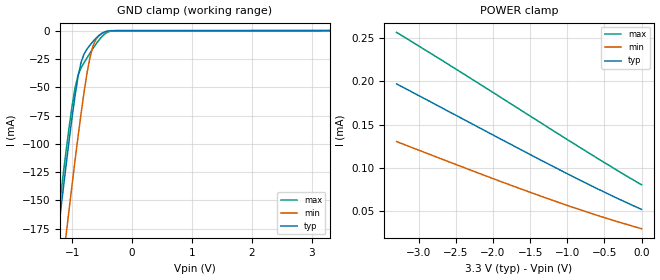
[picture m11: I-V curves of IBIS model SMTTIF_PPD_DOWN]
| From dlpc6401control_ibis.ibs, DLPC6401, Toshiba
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[Model]   SMTTIF_PPD_DOWN
Model_type   Input
Polarity   Non-Inverting
Vinl =   0.8000V
Vinh =   2.0000V
C_comp   1.423pF   NA   NA
|Variable   typ   min   max
[Voltage range]  3.3   3.0   3.6
[Temperature Range]   25.0000   125.000   0.000
[POWER Clamp Reference]   3.3000V   3.0000V   3.6000V
[GND Clamp Reference]   0.000V   0.000V   0.000V
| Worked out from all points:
|   GND clamp passes 1 mA (typ) near -0.45 V on its own axis
[GND_clamp]
| voltage   I(typ)   I(min)   I(max)
-3.3V     -1.18A     -1.24A     -1.166A
-1.3V     -209.3mA   -272.3mA   -195.2mA
-1.25V    -186.1mA   -249mA     -172.2mA
-1.2V     -163.2mA   -225.9mA   -149.6mA
-1.1V     -118.5mA   -180.3mA   -105.8mA
-950mV    -57.05mA   -114.1mA   -50.29mA
-850mV    -27.88mA   -73.01mA   -32.78mA
-700mV    -12.61mA   -23.19mA   -19.66mA
-600mV    -6.597mA   -7.45mA    -11.71mA
-500mV    -2.24mA    -2.388mA   -5.154mA
-300mV    -17.81uA   -59.37uA   -84.02uA
3.3V      52.41uA    37.64uA    66.2uA
[POWER_clamp]
| voltage   I(typ)   I(min)   I(max)
-3.3V     197.1uA    130.6uA    256.5uA
-2.1V     142.7uA    91.1uA     192.6uA
-1.3V     106.7uA    65.95uA    149.2uA
-600mV    76.45uA    45.64uA    111.6uA
0V        52.41uA    30.17uA    80.79uA
